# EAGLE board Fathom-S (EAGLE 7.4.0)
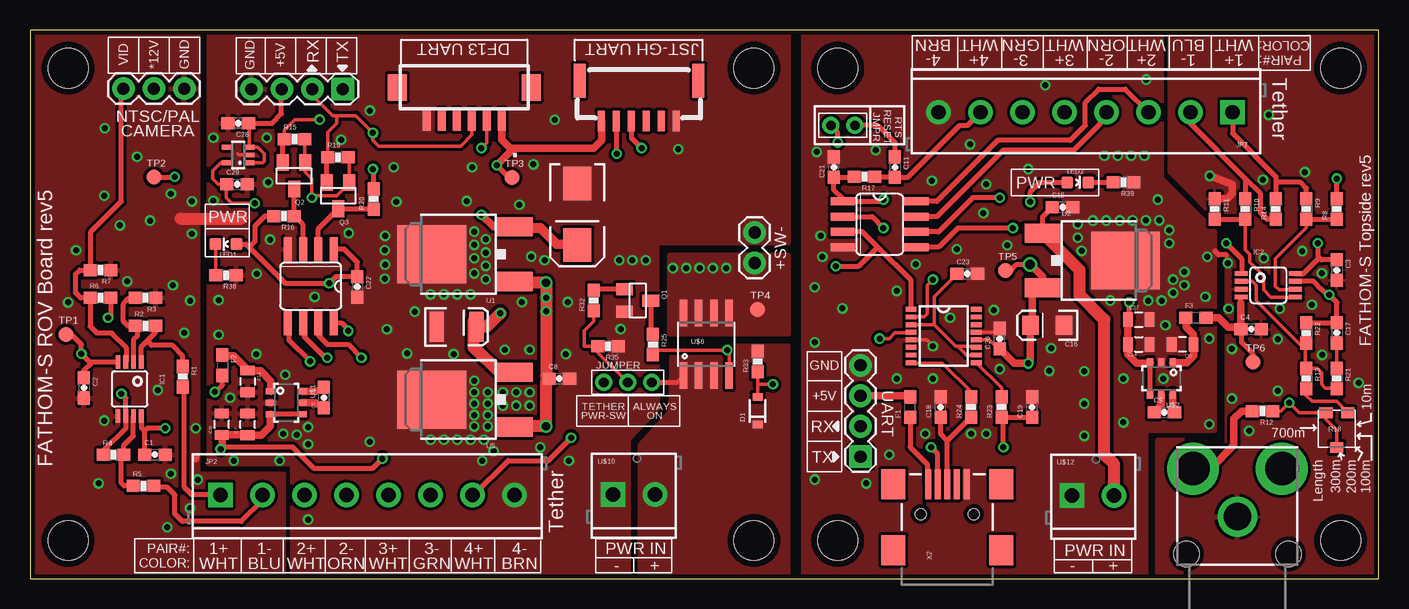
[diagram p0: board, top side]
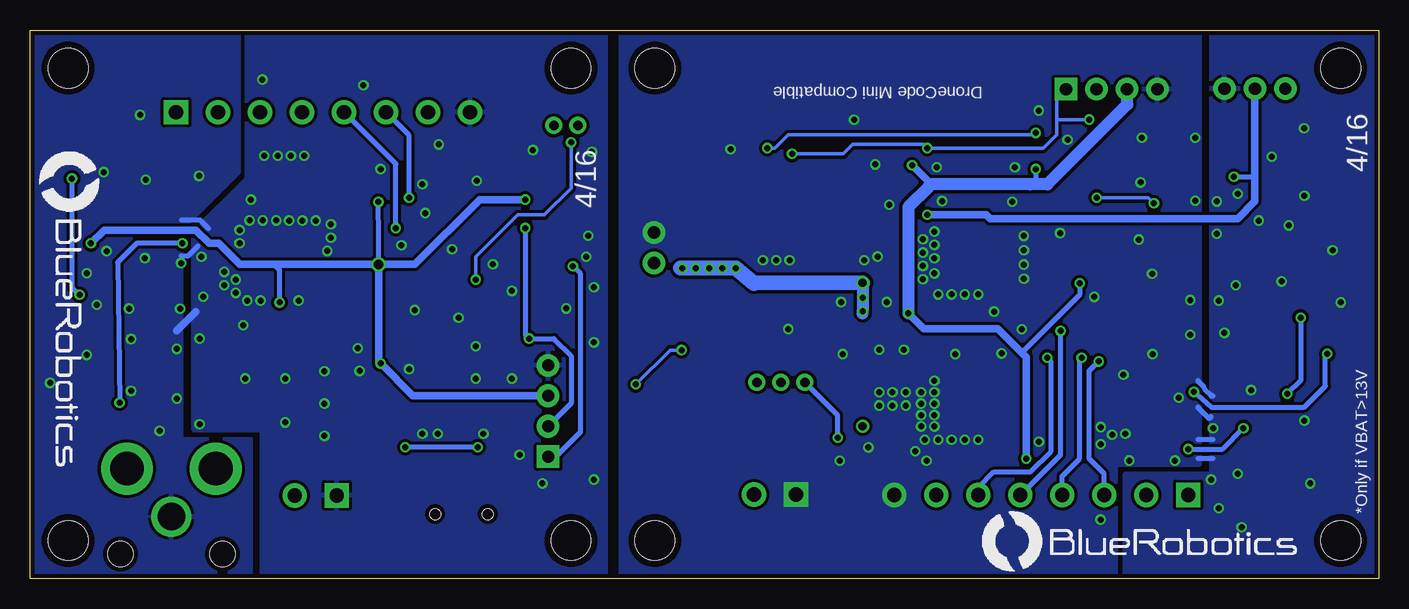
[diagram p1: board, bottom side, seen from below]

Size 112.39 x 45.72 mm. Coordinates in mm from the lower left corner, seen from the top.
Outline: 0,0 112.39,0 112.39,45.72 0,45.72 0,0
Copper layers (1*16): Top 0.0356mm / dielectric 1.5011mm / Bottom 0.0356mm
Design rules "OSH-Park *": minimum track width 6mil, minimum drill 13mil, track to track 6mil, track to pad 6mil, pad to pad 6mil, via to via 6mil, smd to smd 6mil, copper to edge 15mil, drill to drill 6mil, minimum pad ring 7mil, minimum via ring 7mil, stop-mask expansion 3mil, vias tented up to drill 30mil, thermal gap 10mil
Net classes: 1 power: width 0.254 mm

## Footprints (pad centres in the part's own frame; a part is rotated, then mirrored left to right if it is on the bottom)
0603-CAP = smd 1.1 x 1: 1 -0.85,0; 2 0.85,0
0805 = smd 0.8 x 1.2: 1 -0.9,0; 2 0.9,0
EIA3528 = smd 1.2 x 2.5: A 1.65,0; C -1.65,0
C2413 = smd 2.77 x 2.35: + 0,0; - 5.14,0
EIA3216 = smd 1.4 x 1.6: A 1.4,0; C -1.4,0
SOD-323 = smd 0.63 x 0.83: A 1.15,0; C -1.15,0
0603 = smd 1.1 x 1: 1 -0.85,0; 2 0.85,0
MSOP8 = smd 0.4 x 1.1: 1 -0.975,-2.25; 2 -0.325,-2.25; 3 0.325,-2.25; 4 0.975,-2.25; 5 0.975,2.25; 6 0.325,2.25; 7 -0.325,2.25; 8 -0.975,2.25
SO08 = smd 0.66 x 2.032: 1 -1.905,-3.073; 2 -0.635,-3.073; 3 0.635,-3.073; 4 1.905,-3.073; 5 1.905,3.073; 6 0.635,3.073; 7 -0.635,3.073; 8 -1.905,3.073
SSOP16 = smd 0.914 x 0.406: 1 -2.718,2.223; 2 -2.718,1.587; 3 -2.718,0.953; 4 -2.718,0.318; 5 -2.718,-0.318; 6 -2.718,-0.953; 7 -2.718,-1.587; 8 -2.718,-2.223; 9 2.718,-2.223; 10 2.718,-1.587; 11 2.718,-0.953; 12 2.718,-0.318; 13 2.718,0.318; 14 2.718,0.953; 15 2.718,1.587; 16 2.718,2.223
1X04 = drill 1.016 pad 1.88 square: 1 0,0 | drill 1.016 pad 1.88: 2 2.54,0; 3 5.08,0; 4 7.62,0
SCREWTERMINAL-3.5MM-8 = drill 1.2 pad 2.032 square: 1 0,0 | drill 1.2 pad 2.032: 2 3.5,0; 3 7,0; 4 10.5,0; 5 14,0; 6 17.5,0; 7 21,0; 8 24.5,0
1X03 = drill 1.016 pad 1.88: 1 0,0; 2 2.54,0; 3 5.08,0
1X02 = drill 1.016 pad 1.88: 1 0,0; 2 2.54,0
RCA = drill 2.8 pad 4.318: PIN 4,3.7; SWITCH 4,-3.7 | drill 2.3: SHELL 0,0 | hole 2.1: -3.1,4.25; -3.1,-4.25
LED-0603 = smd 1 x 1: A 0,-0.877; C 0,0.877
SOT23 = smd 1 x 1.4: 1 -0.95,-1.1; 2 0.95,-1.1; 3 0,1.1
0603-RES = smd 1.1 x 1: 1 -0.85,0; 2 0.85,0
TRIMPOT_TC33 = smd 1.1 x 0.9: 1 -0.91,-1.45; 2 0,1.45; 3 0.91,-1.45
STAND-OFF = hole 3.302: 0,0
B1,27 = smd 1.27 x 1.27: TP 0,0
DPAK = smd 1.6 x 3: 1 -2.28,-5.31; 3 2.28,-5.31 | smd 4.826 x 5.715: 4 0,1.588
SOT-23-6 = smd 0.51 x 0.8: 1 -0.95,-1.3; 2 0,-1.3; 3 0.95,-1.3; 4 0.95,1.3; 5 0,1.3; 6 -0.95,1.3
DF13C-6P-1.25V = smd 1.6 x 2.2: M$0 5.575,-1.8; M$1 -5.575,-1.8 | smd 0.7 x 1.8: P$1 -3.125,0.9; P$2 -1.875,0.9; P$3 -0.625,0.9; P$4 0.625,0.9; P$5 1.875,0.9; P$6 3.125,0.9
SO08' = smd 0.61 x 2.21: 1 -1.905,-2.616; 2 -0.635,-2.616; 3 0.635,-2.616; 4 1.905,-2.616; 5 1.905,2.616; 6 0.635,2.616; 7 -0.635,2.616; 8 -1.905,2.616
SCREWTERMINAL-3.5MM-2 = drill 1.2 pad 2.032 square: 1 0,0 | drill 1.2 pad 2.032: 2 3.5,0
JST-GH-TOP-6 = smd 0.6 x 1.7: 1 6.25,0; 2 5,0; 3 3.75,0; 4 2.5,0; 5 1.25,0; 6 0,0 | smd 1 x 2.8: MECH1 8.05,-3.35; MECH2 -1.85,-3.35
HEADER-2MM-3POS = drill 0.8 pad 1.422: P$1 0,0; P$2 2,0; P$3 4,0
SC70-5L = smd 0.4 x 0.8: 1 -0.65,-0.95; 2 0,-0.95; 3 0.65,-0.95; 4 0.65,0.95; 5 -0.65,0.95
HEADER-2MM-2POS = drill 0.8 pad 1.422: P$1 0,0; P$2 2,0
USB-MINIB = smd 2.5 x 0.5: D+ 2.5,0; D- 2.5,0.8; GND 2.5,-1.6; ID 2.5,-0.8; VBUS 2.5,1.6 | smd 2.5 x 2: GND@1 -3,-4.5; GND@2 -3,4.5; GND@3 2.5,4.5; GND@4 2.5,-4.5 | hole 0.9: 0,2.2; 0,-2.2

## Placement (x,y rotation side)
C1  0.1uF  [0603-CAP]  10.41,10.34 0 top
C2  0.1uF  [0603-CAP]  4.5,15.9 270 top
C3  0.1uF  [0603-CAP]  108.9,25.72 270 top
C4  0.1uF  [0603-CAP]  101.76,20.8 0 top
C5  1uF X5R 35V  [0603-CAP]  24.5,15.09 90 top
C6  10uF X5R 10V  [0805]  96.04,19.53 180 top
C7  10uF X5R 10V  [0805]  18.14,12.85 90 top
C8  0.1uF  [0603-CAP]  44.12,16.67 0 top
C9  1uF X5R 35V  [0603-CAP]  94.53,13.87 0 top
C10  47uF 10V  [EIA3528]  35.54,21 0 top
C11  1uF  [0603-CAP]  72.07,34.29 270 top
C12  10uF X5R 10V  [0805]  18.14,16.43 270 top
C13  33uF 20V  [C2413]  45.61,27.8 90 top
C14  10uF X5R 10V  [0805]  92.39,19.53 0 top
C15  0.1uF  [0603-CAP]  86.04,30.96 0 top
C16  10uF 16V  [EIA3216]  84.77,21.11 180 top
C17  68pF  [0603-CAP]  108.9,20.48 270 top
C18  47pF  [0603-CAP]  75.88,14.29 90 top
C19  47pF  [0603-CAP]  83.5,14.29 90 top
C20  0.1uF  [0603-CAP]  80.8,20 90 top
C21  0.1uF  [0603-CAP]  66.99,34.29 90 top
C22  0.1uF  [0603-CAP]  27.27,24.31 270 top
C23  0.1uF  [0603-CAP]  78.11,25.4 0 top
C26  10uF X5R 10V  [0805]  15.98,12.87 90 top
C27  10uF X5R 10V  [0805]  92.39,21.59 0 top
C28  1uF  [0603-CAP]  17.35,37.95 180 top
C29  1uF  [0603-CAP]  17.25,32.87 0 top
D1  16V  [SOD-323]  60.63,13.98 90 top
F1  500mA  [0603]  73.34,14.29 90 top
F2  500mA  [0603]  16.03,17.78 270 top
F3  500mA  [0603]  97.16,21.75 0 top
IC1  LMH6643  [MSOP8]  8.31,15.8 180 top
IC2  LMH6643  [MSOP8]  103.19,24.45 270 top
IC3  ST490AB  [SO08]  70.8,29.53 270 top
IC4  ST490AB  [SO08]  23.39,24.37 180 top
IC5  FT230XS  [SSOP16]  76.14,20.22 0 top
JP1  [1X04]  26.06,40.79 180 top
JP2  3.5MM SCREW  [SCREWTERMINAL-3.5MM-8]  15.88,6.99 0 top
JP3  0.1" HEADER  [1X03]  12.86,40.83 180 top
JP5  M02PTH  [1X02]  60.39,28.84 270 top
JP6  PJRAN1X1U04X  [RCA]  100.62,5.17 90 top
JP7  3.5MM SCREW  [SCREWTERMINAL-3.5MM-8]  100.22,38.87 180 top
JP15  0.1" HEADER  [1X04]  69.22,10.16 90 top
LED1  GREEN  [LED-0603]  16.33,27.88 90 top
LED2  GREEN  [LED-0603]  87.31,33.02 270 top
Q1  BC817-40W  [SOT23]  50.64,23.18 270 top
Q2  BSS138  [SOT23]  22,33.57 180 top
Q3  BSS138  [SOT23]  25.67,31.91 180 top
R1  43  [0603-RES]  12.73,16.83 270 top
R2  3K  [0603-RES]  9.61,21.06 0 top
R3  3K  [0603-RES]  9.64,23.39 180 top
R4  3K  [0603-RES]  6.97,10.31 0 top
R5  43  [0603-RES]  9.46,7.72 0 top
R6  1.5K  [0603-RES]  5.87,23.39 0 top
R7  75  [0603-RES]  5.87,25.72 180 top
R8  3K  [0603-RES]  108.9,30.8 90 top
R9  3K  [0603-RES]  106.36,30.8 270 top
R10  3K  [0603-RES]  101.28,30.8 270 top
R11  3K  [0603-RES]  98.74,30.8 270 top
R12  75  [0603-RES]  102.71,13.97 180 top
R13  1.5K  [0603-RES]  106.36,16.67 270 top
R14  86.6  [0603-RES]  103.82,30.8 90 top
R15  10K  [0603-RES]  22.03,36.63 0 top
R16  10K  [0603-RES]  21.16,30.22 180 top
R17  47K  [0603-RES]  69.53,33.5 180 top
R18  TC33X-2-102E  [TRIMPOT_TC33]  108.9,12.38 180 top
R19  10K  [0603-RES]  25.67,35.12 0 top
R20  10K  [0603-RES]  28.63,31.62 90 top
R21  3.9K  [0603-RES]  108.9,16.67 270 top
R22  3K  [0603-RES]  106.36,20.48 270 top
R23  27  [0603-RES]  80.96,14.29 90 top
R24  27  [0603-RES]  78.42,14.29 90 top
R25  10K  [0603-RES]  51.91,19.53 270 top
R32  47K  [0603-RES]  46.99,23.18 90 top
R33  5.1K  [0603-RES]  60.64,18.1 90 top
R35  47K  [0603-RES]  48.18,19.37 180 top
R38  330  [0603-RES]  16.32,25.29 180 top
R39  330  [0603-RES]  91.12,33.02 180 top
STANDOFF1  STAND-OFF  [STAND-OFF]  3.17,3.17 0 top
STANDOFF2  STAND-OFF  [STAND-OFF]  60.33,3.17 0 top
STANDOFF3  STAND-OFF  [STAND-OFF]  60.33,42.55 0 top
STANDOFF4  STAND-OFF  [STAND-OFF]  3.17,42.55 0 top
STANDOFF5  STAND-OFF  [STAND-OFF]  67.31,3.17 0 top
STANDOFF6  STAND-OFF  [STAND-OFF]  109.22,3.17 0 top
STANDOFF7  STAND-OFF  [STAND-OFF]  67.31,42.55 0 top
STANDOFF8  STAND-OFF  [STAND-OFF]  109.22,42.55 0 top
TP1  -5V  [B1,27]  2.98,20.35 0 top
TP2  12V  [B1,27]  10.32,33.45 0 top
TP3  5V  [B1,27]  40.16,33.42 0 top
TP4  VIN  [B1,27]  60.64,22.43 0 top
TP5  5V  [B1,27]  81.28,25.67 0 top
TP6  -5V  [B1,27]  101.92,18.05 0 top
U1  MC7812  [DPAK]  35.07,27.04 90 top
U2  MC7805  [DPAK]  89.69,26.51 270 top
U5  MC7805  [DPAK]  35.07,14.92 90 top
U$1  LM2776  [SOT-23-6]  21.36,14.66 270 top
U$2  LM2776  [SOT-23-6]  94.28,16.68 180 top
U$3  DF13-6P-1.25V  [DF13C-6P-1.25V]  36.19,39.14 180 top
U$4  LOGOFULL-M  [BR-FULL-LOGO-MEDIUM]  35.08,-0.79 0 bottom
U$5  LOGOBR-LOGO-MS-COPPER  [BR-LOGO-MEDIUM-SMALL-COPPER]  110.31,34.32 90 top
U$6  AO4407A  [SO08']  56.36,19.53 0 top
U$7  LOGOFULL-M  [BR-FULL-LOGO-MEDIUM]  113.03,37.62 270 bottom
U$9  LOGOBR-LOGO-MS  [BR-LOGO-MEDIUM-SMALL-COPPER]  51.1,33.56 270 top
U$10  M023.5MM  [SCREWTERMINAL-3.5MM-2]  48.58,7 0 top
U$11  JST-GH-6TOP-ENTRY  [JST-GH-TOP-6]  53.86,38.14 180 top
U$12  M023.5MM  [SCREWTERMINAL-3.5MM-2]  86.84,6.94 0 top
U$13  HEADER-33MM  [HEADER-2MM-3POS]  47.81,16.35 0 top
U$15  VREG-MIC5365  [SC70-5L]  17.34,35.3 90 top
U$16  HEADER-22MM  [HEADER-2MM-2POS]  68.74,37.77 180 top
X2  USBSMD  [USB-MINIB]  76.44,5.38 90 top

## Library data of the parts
C1-C10 C12 C14-C17 C26-C29 R1-R14 R21 R22 = SparkFun-Passives
C11 C18-C23 F1-F3 R15-R17 R19 R20 R23 R24 X2 = SparkFun
C13 IC1 IC2 JP6 TP1-TP6 U$4 U$5 U$7 U$9 U$13 U$15 U$16 = BlueRobotics-Main
D1 = SparkFun-DiscreteSemi; PROD_ID: DIO-11284; VALUE: 3.3V
IC3 IC4 = maxim; MF: MAXIM; MPN: MAX488CSA; OC_FARNELL: 3534170; OC_NEWARK: 34C3921
IC5 = ftdichip
JP1-JP3 JP5 JP7 JP15 U$10 U$12 = SparkFun-Connectors
LED1 LED2 = SparkFun-LED
Q1 U$6 = SparkFun-DiscreteSemi
Q2 Q3 = SparkFun-DiscreteSemi; PROD_ID: TRANS-00830
R18 STANDOFF1-STANDOFF8 = SparkFun-Electromechanical
R25 R32 R33 R35 R38 R39 = SparkFun-Resistors
U1 U2 U5 U$1 U$2 = BR-Eagle-Library
U$3 = con-hirose-df13
U$11 = BlueRobotics-JST-GH

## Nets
3.3V-ISO: C29.1 Q2.1 Q3.1 R15.2 R19.2 U$15.5
3V3OUT: C23.1 IC5.3 IC5.10 IC5.11
12V-ISO: C13.+ JP3.2 TP2.TP U1.3
-VCC: C4.1 F3.2 IC2.4 TP6.TP
-VCC-ISO: C2.1 F2.2 IC1.4 TP1.TP
-VCC-ISO-PRE: C12.1 F2.1 U$1.1
-VCC-PRE: C6.1 F3.1 U$2.1
CAMERA: IC1.3 JP3.3 R6.1 R7.2
GND: C3.2 C4.2 C6.2 C14.2 C15.2 C16.C C18.2 C19.2 C20.2 C21.2 C23.2 C27.2 IC2.3 IC3.4 IC5.5 IC5.13 JP6.SHELL JP7.8 JP15.4 R11.1 R39.1 U2.4 U$2.2 U$12.1 X2.GND
GND-ISO: C1.2 C2.2 C7.2 C8.2 C10.C C12.2 C13.- C22.2 C26.2 C28.2 C29.2 IC1.5 IC4.4 JP1.4 JP2.8 JP3.1 JP5.1 Q1.2 R3.1 R7.1 R35.1 R38.1 U1.4 U5.4 U$1.2 U$3.P$6 U$10.1 U$11.6 U$15.2
N$1: IC1.1 R1.1 R2.2
N$2: IC1.7 R4.2 R5.1
N$3: C9.1 U$2.5
N$4: C9.2 U$2.6
N$5: IC1.2 R2.1 R3.2
N$6: IC1.6 R4.1 R6.2
N$7: C11.1 U$16.P$1
N$8: IC2.5 R10.2 R11.2
N$9: IC2.6 R8.1 R9.2
N$10: C5.1 U$1.5
N$11: C5.2 U$1.6
N$12: R13.2 R18.1
N$14: C17.1 IC2.7 R8.2 R22.1
N$15: IC2.2 R13.1 R21.2 R22.2
N$16: C17.2 R21.1
N$17: IC2.1 R12.1 R18.2 R18.3
N$19: C19.1 R23.1 X2.D-
N$20: C18.1 R24.1 X2.D+
N$21: F1.1 X2.VBUS
N$22: IC5.8 R24.2
N$27: Q1.1 R32.2
N$28: D1.A R25.2 R33.1 U$6.4
N$29: IC5.9 R23.2
N$30: Q1.3 R25.1
N$31: LED1.C R38.2
N$32: LED2.C R39.2
ROV-BATT: D1.C R33.2 U$6.1 U$6.2 U$6.3 U$10.2 U$13.P$3
ROV-ON: JP2.7 U$13.P$1
ROV-ON-CTRL: C11.2 JP7.7 R17.1
ROV-ON-SELECT: R32.1 R35.2 U$13.P$2
ROV-RX: IC4.2 Q3.3 R20.1
ROV-TP1+: JP2.1 R1.2
ROV-TP1-: JP2.2 R5.2
ROV-TP2+: IC4.5 JP2.3
ROV-TP2-: IC4.6 JP2.4
ROV-TP3+: IC4.8 JP2.5
ROV-TP3-: IC4.7 JP2.6
ROV-TX: IC4.3 Q2.3 R16.1
ROV-VIN: C8.1 JP5.2 TP4.TP U1.1 U5.1 U$6.5 U$6.6 U$6.7 U$6.8
RTS: IC5.2 U$16.P$2
RX-3.3V: JP1.2 Q3.2 R19.1 U$3.P$3 U$11.3
RX-I: IC3.2 IC5.4 JP15.2
TOP-TP1+: JP7.1 R9.1 R14.2
TOP-TP1-: JP7.2 R10.1 R14.1
TOP-TP2+: IC3.8 JP7.3
TOP-TP2-: IC3.7 JP7.4
TOP-TP3+: IC3.5 JP7.5
TOP-TP3-: IC3.6 JP7.6
TOP-VIN: C15.1 U2.1 U$12.2
TX-3.3V: JP1.1 Q2.2 R15.1 U$3.P$2 U$11.2
TX-O: IC3.3 IC5.1 JP15.1
VCC: C3.1 C14.1 C16.A C20.1 C21.1 C27.1 F1.2 IC2.8 IC3.1 IC5.12 JP15.3 LED2.A R17.2 TP5.TP U2.3 U$2.3 U$2.4
VCC-ISO: C1.1 C7.1 C10.A C22.1 C26.1 C28.1 IC1.8 IC4.1 JP1.3 LED1.A R16.2 R20.2 TP3.TP U5.3 U$1.3 U$1.4 U$3.P$1 U$11.1 U$15.1 U$15.3
VIDEO-OUT: JP6.PIN R12.2

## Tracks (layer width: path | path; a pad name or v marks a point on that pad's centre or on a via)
3.3V-ISO  (via drill 0.5)
  Top 0.305: U$15.5 16.4,34.64 15.91,34.64 15.24,33.97 15.24,33.34 15.71,32.87 C29.1 16.35,32.82 16.35,31.75 16.83,31.27 v18.73,31.27 | R15.2 22.88,34.74 Q2.1 22.95,33.88 23.5,33.34 v23.5,31.75 23.81,31.91 25.56,31.91 26.62,32.97 Q3.1 26.62,35.02 R19.2
  Bottom 0.305: v23.5,31.75 19.21,31.75 v18.73,31.27
3V3OUT
  Top 0.305: IC5.3 75.35,21.17 | 75.35,21.17 77.15,19.37 77.31,19.37 | 77.31,19.37 78.75,19.37 IC5.11 | IC5.10 78.05,18.63 77.31,19.37 | 75.35,21.17 75.35,23.49 C23.1
12V-ISO  (via drill 0.5)
  Top 0.406: TP2.TP 12.02,33.45 v12.06,33.5
  Top 0.61: U1.3 38.63,29.32 v37.62,30.32
  Top 0.813: C13.+ 43.88,27.88 42.55,29.21 40.48,29.21 U1.3
  Bottom 0.406: v12.06,33.5 10.48,33.5 10.32,33.66
  Bottom 0.61: JP3.2 10.32,33.66 10.32,31.43 11.75,30 32.38,30 32.7,30.32 v37.62,30.32
-VCC
  Top 0.406: 100.89,22.94 100.89,23.42 IC2.4 | TP6.TP 101.92,18.73 100.97,19.68 100.97,20.74
  Top 0.61: C4.1 100.91,22.92 100.89,22.94 | 100.97,20.74 C4.1 | F3.2 99.06,21.75 99.85,20.95 100.75,20.95 C4.1
-VCC-ISO  (via drill 0.5)
  Top 0.406: v4.29,18.73 4.29,18.57 | IC1.4 5.18,18.05 | 5.18,18.05 4.97,18.05 v4.29,18.73 | C2.1 4.5,17.36 5.18,18.05 | v15.4,15.56 16.03,16.14 F2.2 | v4.29,18.73 4.29,19.53 3.65,20.16 3.18,20.16 TP1.TP
  Bottom 0.406: v4.29,18.73 4.45,18.57 4.45,16.03 6.19,14.29 13.97,14.29 v15.4,15.56
-VCC-ISO-PRE
  Top 0.61: U$1.1 20.06,16.45 19.21,17.3 18.17,17.3 C12.1 18.14,17.42 16.99,18.57 16.09,18.57 F2.1
-VCC-PRE
  Top 0.61: F3.1 96.36,21.69 96.36,20.95 96.94,20.37 C6.1 97,19.47 97,18.57 96.4,17.98 U$2.1
CAMERA
  Top 0.406: R7.2 4.13,25.72 3.81,25.4 3.81,23.81 4.23,23.39 R6.1 5.02,21.02 5.56,20.48 6.83,20.48 6.83,20.45 8,19.28 8,18.07 IC1.3 | 5.08,25.78 5.08,28.89 7.62,31.43 7.62,40.67 JP3.3
  Top 0.61: 5.08,25.78 R7.2
GND  (via drill 0.5)
  Top 0.305: IC5.5 74.71,19.9 v75.25,19.37 | IC5.13 80.97,20.54 C20.2
  Top 0.406: 99.69,26.99 99.06,26.99 98.74,27.3
  Top 0.61: R11.1 99.75,31.65 100.17,32.07 100.17,32.89 v98.3,33.56
  Bottom 0.406: 99.82,26.9 99.21,26.9 98.37,27.74 | 97.53,29.18 98.22,29.88 99.75,29.88
  Bottom 0.61: 100.17,20.64 98.58,22.23
  other vias: 80.33,22.38 75.25,16.67 94.61,21.11 94.46,16.67 91.12,13.02 106.83,22.82 100.16,15.01 110.72,16.31 103.23,38.64 102.75,33.24 95.25,24.92 94.93,29.05 93.98,31.59 106.01,27.3 107.66,25.45 84.93,17.3 79.69,12.06 72.23,16.67 72.23,23.97 65.41,24.29 65.56,35.56 73.82,26.19 76.68,21.75 85.09,19.21 90.81,29.84 87.31,28.42 81.44,27.78 66.04,26.83 98.11,26.83 91.12,16.67 74.61,12.06 65.41,8.26 83.19,34.13 93.03,41.59 84.61,41.12 70.48,35.72 80.8,17.46 65.88,28.57 65.41,19.68 69.69,7.94 71.6,10.32 107.67,18.64 101.59,12.31 106.24,33.88 97.95,23.5 78.42,12.06 103.97,19.96 103.97,15.65 100.16,19.14 99.89,22.49 99.81,26.3 102.81,26.71 104.14,22.5 90.01,23.18 93.19,23.18 98.27,20 91.88,29.85 92.99,29.85 94.1,29.85 89.69,29.84 88.58,29.84 87.31,29.53 87.63,27.3 94.93,27.94 95.25,23.81 94.3,23.18 96.2,24.45 96.2,25.56 98.27,12.86 89.53,35.24 90.65,35.24 91.76,35.24 92.87,35.24 79.45,30.47 77.23,27.45 75.16,33.17 78.34,36.18 87.86,17.29 87.86,14.59 87.86,11.89 79.7,32.87 67.7,22.51
  pour Top (isolate 0.254): 99.69,0 99.69,29.05 94.93,33.81 94.93,45.72 114.3,45.72 114.3,0
  pour Bottom (isolate 0.254): 99.69,-2.54 99.69,29.05 94.93,33.81 94.93,48.26 112.39,48.26 112.39,-2.54
  pour Bottom (isolate 0.254): 64.45,-2.54 93.03,-2.54 93.03,12.38 98.74,12.38 98.74,28.89 94.3,33.34 94.3,48.26 64.45,48.26
  pour Top (isolate 0.254, no thermals): 64.45,-1.27 93.03,-1.27 93.03,12.38 98.74,12.38 98.74,28.89 94.3,33.34 94.3,48.26 64.45,48.26
  pour Bottom (isolate 0.254): 93.98,-1.27 93.98,11.59 101.6,11.59 101.6,-1.27
  pour Top (isolate 0.254): 93.98,-2.54 93.98,11.59 101.6,11.59 101.6,-2.54
GND-ISO  (via drill 0.5)
  Top 0.305: U$15.2 17.4,35.3 17.3,35.4
  Top 0.61: 13.81,10.16 13.81,10
  Top 1.016: 12.54,30 17.62,30
  Bottom 0.406: 13.97,13.49 14.13,13.34 15.08,14.29 | 13.81,15.24 13.97,15.24 14.45,15.72 14.61,16.03 15.08,16.51 | 13.81,10 15.08,10 | 13.81,11.59 15.08,11.59
  other vias: 49.21,20.8 40.78,31.16 30.54,31.41 31.43,18.76 13.49,28.73 13.49,31.43 10.64,15.72 11.43,4.29 5.71,7.94 6.19,13.18 3.17,23.02 12.86,20.48 6.19,31.91 16.67,15.08 21.27,16.99 21.11,12.06 15.72,20.32 13.34,23.18 19.84,33.02 18.89,25.4 29.58,26.17 29.58,28.56 44.81,23.05 35.3,18.71 33.38,11.57 34.49,11.57 44.67,18.71 49.09,26.54 37.98,27.17 23.18,4.92 13.34,5.87 13.97,8.26 13.81,12.54 30.32,34.29 37.68,9.82 38.63,10.62 40.52,15.54 40.52,14.43 39.41,15.54 39.41,14.43 35.6,11.57 37.98,26.06 37.98,24.95 41,23.05 20.8,9.84 16.99,9.84 15.71,23.21 11.75,8.73 11.91,24.45 8.1,24.77 20,28.26 29.57,27.37 29.57,24.99 26.56,28.8 23.71,23.48 29.74,20.78 32.06,22.26 37.98,28.29 38.14,15.54 37.03,14.59 38.14,14.59 37.03,13.63 37.03,16.49 37.03,15.54 38.14,13.63 38.14,12.68 37.03,12.68 41.63,15.54 41.63,14.43 37.03,28.92 37.03,27.81 37.03,26.7 37.03,25.43 33.38,23.68 34.49,23.68 35.6,23.68 36.71,23.68 36.39,31.46 39.57,19.08 41.63,19.08 28.31,11.41 22.22,12 23.17,12.63 23.17,11.21 36.71,11.57 37.82,11.57 8.92,35.15 7.49,29.44 6.22,37.53 3.84,27.37 10,29.84 11.75,32.07 18.85,18.72 19.73,36.74 25.93,36.58 15.29,36.74 15.29,31.5 36.83,34.28 43.72,38.23 41.95,34.52 54.02,35.79 28.32,39.01 42.53,10.94 44.91,9.83 42.88,26.53 41.77,26.84 50.21,26.54 51.32,26.54
  pour Top (isolate 0.254): 12.7,-3.33 12.7,8.75 21.11,8.75 21.11,-3.33
  pour Bottom (isolate 0.254, no thermals): 21.91,45.72 63.18,45.72 63.18,-5.08 21.91,-5.08
  pour Top (isolate 0.254, no thermals): 21.91,48.26 63.18,48.26 63.18,27.94 52.23,27.94 52.23,25.08 52.26,23.34 52.26,14.18 49.85,11.64 49.85,-2.54 21.91,-2.54
  pour Top (isolate 0.254): 13.97,-1.27 -1.27,-1.27 -1.27,46.99 13.97,46.99
  pour Bottom (isolate 0.254): 13.97,-2.54 0,-2.54 0,48.26 13.97,48.26
  pour Bottom (isolate 0.254): 21.11,8.73 13.34,8.73 13.34,0 21.11,0
  pour Bottom (isolate 0.254): 14.92,9.53 14.92,46.99 27.29,46.99 27.29,9.53
  pour Top (isolate 0.254): 14.92,9.53 14.92,48.26 24.13,48.26 24.13,9.53
N$1
  Top 0.406: R1.1 12.72,18.59 11.89,19.43 10.13,19.43 9.75,19.81 | 10.21,20.8 R2.2 10.44,21.03 10.44,20.5 9.75,19.81 | IC1.1 9.28,19.34 9.75,19.81
N$2
  Top 0.406: R5.1 7.84,7.72 7.62,7.94 7.62,10.11 R4.2 7.82,11.1 8.61,11.89 8.61,13.53 IC1.7
N$3
  Top 0.61: U$2.5 94.28,14.48 C9.1
N$4
  Top 0.61: U$2.6 95.23,14.01 C9.2
N$5
  Top 0.406: R3.2 8.73,23.34 8.17,23.34 7.78,22.87 7.78,21.43 8.15,21.06 R2.1 8.94,20.88 8.94,20.22 8.61,19.89 8.61,18.07 IC1.2
N$6  (via drill 0.5)
  Top 0.406: R6.2 6.72,21.96 v6.51,21.75 | R4.1 6.12,10.69 8,12.57 8,13.53 IC1.6 7.98,15.04 v7.62,15.4
  Bottom 0.406: v6.51,21.75 6.51,16.51 v7.62,15.4
N$7
  Top 0.406: C11.1 72.07,36.35 70.64,37.78 68.76,37.78 U$16.P$1
N$8
  Top 0.305: R10.2 101.28,27.42 101.65,27.05 101.65,26.36 102.79,25.22 102.79,24.08 103.4,23.47 IC2.5
  Top 0.406: R11.2 R10.2
N$9
  Top 0.305: R9.2 106.36,29.25 103.78,26.67 103.78,24.38 104.09,24.08 105.39,24.08 IC2.6
  Top 0.406: R9.2 R8.1
N$10
  Top 0.61: U$1.5 23.76,14.66 C5.1
N$11
  Top 0.61: U$1.6 23.85,15.61 C5.2
N$12
  Top 0.305: R13.2 106.36,15.24 106.84,14.76 108.88,14.76 R18.1
  Top 0.406: 110.01,13.95 R18.1
N$14  (via drill 0.5)
  Top 0.406: R8.2 v108.9,33.34 | R22.1 C17.1 108.9,23.02 v108.27,23.65 108.1,23.65 107.62,24.13 | 107.63,24.13 107.62,24.13 | 107.62,24.13 106.98,24.77 IC2.7
  Bottom 0.406: v108.9,33.34 108.9,24.29 v108.27,23.65
N$15
  Top 0.305: IC2.2 101.87,24.77 102.18,24.46 102.18,23.16 105.82,19.53 106.26,19.53 106.26,17.62 R13.1 107.26,17.52 107.63,17.14 107.63,16.19 107.95,15.88 108.85,15.88 R21.2
  Top 0.406: 106.26,19.53 R22.2
N$16
  Top 0.305: C17.2 R21.1
N$17  (via drill 0.5)
  Top 0.305: R18.2 108.9,12.38 107.99,13.29 R18.3 105.76,13.83 v104.93,14.66 104.25,13.97 R12.1
  Top 0.406: v99.69,27.94 100.97,26.67 100.97,25.45 IC2.1 | 104.93,14.92 v104.93,14.66 | 108.88,10.95 R18.2
  Bottom 0.406: v99.69,27.94 103.5,27.94 105.09,26.35 v104.93,14.66
N$19  (via drill 0.5)
  Top 0.406: X2.D- 75.64,10.4 v75.09,10.95 | v81.12,10.95 81.12,13.28 R23.1 C19.1
  Bottom 0.406: v75.09,10.95 v81.12,10.95
N$20
  Top 0.406: X2.D+ 76.44,11.5 | 76.44,11.5 75.88,12.06 C18.1 | R24.1 78.38,13.44 76.44,11.5
N$21
  Top 0.406: F1.1 73.34,10.95 74.77,9.53 74.77,7.96 X2.VBUS
N$22
  Top 0.305: R24.2 78.42,15.56 76.04,17.94 73.48,17.94 IC5.8
N$27
  Top 0.406: Q1.1 47.25,24.13 R32.2
N$28  (via drill 0.5)
  Top 0.305: R33.1 60.64,16.19 | 60.64,16.19 60.64,15.47 D1.A | v61.91,16.19 60.64,16.19 | R25.2 52.28,19.05 v58.1,19.05 58.26,18.89 U$6.4
  Bottom 0.305: v58.1,19.05 59.05,19.05 v61.91,16.19
N$29
  Top 0.305: R23.2 80.96,15.89 IC5.9
N$30
  Top 0.406: Q1.3 51.74,20.39 R25.1
N$31
  Top 0.305: R38.2 15.47,27.86 LED1.C
N$32
  Top 0.406: LED2.C R39.2
ROV-BATT
  Top 0.305: 53.89,16.35 U$6.1
  Top 0.406: U$13.P$3 53.89,16.35
  pour Top (isolate 0.254, no thermals): 50.8,-2.54 63.18,-2.54 63.18,19.37 53.5,19.37 53.34,13.97 50.8,11.11
ROV-ON  (via drill 0.5)
  Top 0.406: JP2.7 36.99,6.99 39.85,9.84 43.18,9.84 v45.09,11.75
  Bottom 0.406: v45.09,11.75 45.09,13.62 U$13.P$1
ROV-ON-CTRL
  Top 0.406: JP7.7 78.14,37.78 77.47,37.78 73.13,33.44 C11.2 72.02,33.5 R17.1
ROV-ON-SELECT
  Top 0.305: R32.1 46.99,21.43 46.2,20.64 46.2,19.37 R35.2 47.33,18.84 U$13.P$2
ROV-RX
  Top 0.406: IC4.2 24.03,29.17 Q3.3 28.58,30.82 R20.1
ROV-TP1+
  Top 0.406: JP2.1 13.49,6.99 12.86,7.62 12.86,15.84 R1.2
ROV-TP1-
  Top 0.406: JP2.2 19.38,6.52 17.62,4.76 12.7,4.76 12.06,5.4 12.06,6.99 11.43,7.62 10.41,7.62 R5.2
ROV-TP2+  (via drill 0.5)
  Top 0.406: v23.34,18.1 21.59,19.84 21.59,21.2 IC4.5
  Bottom 0.406: JP2.3 22.88,8.75 24.13,10 24.13,17.3 v23.34,18.1
ROV-TP2-  (via drill 0.5)
  Top 0.406: v24.77,18.41 24.61,18.41 22.86,20.16 22.86,21.2 IC4.6
  Bottom 0.406: JP2.4 26.38,8.55 24.92,10 24.92,18.26 v24.77,18.41
ROV-TP3+  (via drill 0.5)
  Top 0.406: v26.51,20.64 26.51,20.8 26.04,21.27 25.33,21.27 IC4.8
  Bottom 0.406: JP2.5 29.84,6.99 26.51,10.32 v26.51,20.64
ROV-TP3-  (via drill 0.5)
  Top 0.406: IC4.7 24.03,20.26 24.77,19.53 26.51,19.53 v27.62,18.41
  Bottom 0.406: JP2.6 33.38,7.58 32.07,8.89 29.05,8.89 27.3,10.64 27.3,18.1 v27.62,18.41
ROV-TX
  Top 0.406: IC4.3 22.76,29.47 R16.1 22.01,32.46 Q2.3
ROV-VIN  (via drill 0.5, 0.7)
  Top 1.016: U1.1 40.48,24.65 v43.01,24.65 43.01,16.93 C8.1 43.01,16.41 v43.01,12.7 40.44,12.7 U5.1 | v43.01,23.42 v43.01,22.28
  Bottom 1.016: v43.01,24.65 v43.01,22.27 | 43.01,22.11 v43.01,22.27 | v43.01,22.27 v43.01,22.28
  Bottom 1.27: v43.01,24.65 52.07,24.61 v53.58,25.88 58.18,25.88
  other vias: 54.69,25.88 55.8,25.88 56.91,25.88 58.02,25.88
  pour Top (isolate 0.254, no thermals): 53.32,20.36 53.32,27 63.18,26.99 63.18,20.32
RTS  (via drill 0.5)
  Top 0.305: IC5.2 74.51,21.81 74.77,22.07 74.77,24.45 v75.25,24.92
  Top 0.406: v67.31,36.35 67.31,37.19 U$16.P$2
  Bottom 0.305: v75.25,24.92 75.25,26.83 71.75,30.32 69.53,30.32 67.31,32.54 v67.31,36.35
RX-3.3V  (via drill 0.5)
  Top 0.305: U$3.P$3 36.81,36.97 35.88,36.04 29.05,36.04 28.57,36.51 v28.57,37.15 27.15,38.58 25.56,38.58 | JP1.2 23.52,40.29 25.24,38.58 25.56,38.58 | R19.1 24.82,37.2 25.56,37.94 25.56,38.58
  Top 0.406: U$11.3 50.11,36.73 v50.96,35.88 | Q3.2 24.72,35.03 R19.1
  Bottom 0.305: v50.96,35.88 50.32,35.88 49.21,36.99 28.73,36.99 v28.57,37.15
RX-I  (via drill 0.5)
  Top 0.305: v70.8,20 71.6,20 72.07,20.48 73.36,20.48 IC5.4
  Top 0.406: IC3.2 70.17,30.16 v71.12,29.21
  Bottom 0.406: v71.12,29.21 71.12,20.32 v70.8,20 68.74,20 67.31,18.57 67.31,14.61 JP15.2
TOP-TP1+
  Top 0.406: JP7.1 100.22,37.1 103.82,33.5 103.82,33.18 | 103.82,33.18 R14.2 | R9.1 106.36,32.54 105.89,33.02 103.98,33.02 103.82,33.18
TOP-TP1-
  Top 0.406: JP7.2 96.72,37.9 101.28,33.34 | 101.28,33.34 R10.1 | R14.1 103.08,29.95 102.55,30.48 102.55,32.07 101.28,33.34
TOP-TP2+
  Top 0.406: JP7.3 91.29,40.8 89.06,40.8 87.95,39.69 87.95,37.78 86.68,36.51 80.64,36.51 75.56,31.43 IC3.8
TOP-TP2-
  Top 0.406: JP7.4 89.22,38.36 89.22,37.94 87,35.72 81.12,35.72 75.56,30.16 IC3.7
  Bottom 0.406: 89.69,38.84 JP7.4
TOP-TP3+  (via drill 0.5)
  Top 0.406: v81.92,29.21 77.31,29.21 75.72,27.62 IC3.5
  Bottom 0.406: JP7.5 81.92,34.56 v81.92,29.21
TOP-TP3-  (via drill 0.5)
  Top 0.406: v80.8,31.75 78.58,31.75 75.72,28.89 IC3.6
  Bottom 0.406: JP7.6 80.8,36.95 v80.8,31.75
TOP-VIN
  Top 0.406: U2.1 84.38,30.15 C15.1
  Top 1.016: U2.1 87.47,25.7 87.47,23.65 89.53,21.59 89.53,10.32 90.34,9.52 U$12.2
TX-3.3V  (via drill 0.5)
  Top 0.305: U$3.P$2 38.06,36.32 v37.62,35.88 | R15.1 21.18,37.37 22.07,38.26 v24.13,38.26
  Top 0.406: U$11.2 48.86,35.44 v48.9,35.4 | Q2.2 21.05,36.5 R15.1
  Bottom 0.305: v48.9,35.4 44.61,35.4 43.81,36.2 37.94,36.2 v37.62,35.88 27.94,35.88 26.83,36.99 26.83,38.1 | 26.83,38.1 26.83,40.03 JP1.1 | v24.13,38.26 26.67,38.26 26.83,38.1
TX-O  (via drill 0.5)
  Top 0.406: IC5.1 73.42,24.85 70.64,27.62 | 70.64,27.62 69.37,28.89 IC3.3 | v67.15,26.04 69.06,26.04 70.64,27.62
  Bottom 0.406: JP15.1 68.58,10.16 66.52,12.22 66.52,25.4 v67.15,26.04
VCC  (via drill 0.5, 0.8)
  Top 0.305: IC5.12 79.95,19.9 80.64,19.21 81.22,19.21 C20.1
  Top 0.406: C3.1 107.63,26.57 107.45,26.75 | v107.31,27.94 107.31,26.89 107.45,26.75 | v71.12,31.59 71.28,31.43 IC3.1 67.73,31.65 66.99,32.38 C21.1 68.63,33.44 R17.2 | U$2.4 U$2.3 | IC2.8 106.12,25.42 107.45,26.75 | 91.6,21.7 v91.6,23.02 | v83.36,31.39 83.36,32.24 84.14,33.02 LED2.A | TP5.TP 81.71,25.67 82.23,26.19 v83.34,26.19
  Top 0.61: JP15.3 72.89,15.24 F1.2 | C20.1 82.02,17.94 v83.19,17.94 83.37,18.13 C16.A 83.37,20.98 | 91.44,19.47 C14.1 | 91.6,19.63 C14.1 | 91.6,21.7 C27.1 C14.1 | C14.1 91.49,18.68 92.23,17.94 93.29,17.94 U$2.3 | U2.3 84.38,25.15 v83.34,26.19 | 83.5,24.13 83.5,21.11 83.37,20.98 | 83.37,20.98 83.34,20.95
  Bottom 0.406: v83.34,26.19 83.34,28.36 v83.36,31.39 | v91.6,23.02 91.6,25.72 92.08,26.19
  Bottom 0.61: v107.31,27.94 106.2,29.05 98.58,29.05 97.47,27.94 96.68,27.94 94.93,26.19 92.08,26.19 v83.34,26.19 | JP15.3 80.49,15.24 v83.19,17.94 83.34,18.1 v83.34,26.19 | v83.34,26.19 80.33,26.19 74.93,31.59 v71.12,31.59
VCC-ISO  (via drill 0.5)
  Top 0.305: U$15.1 19.41,34.65 19.53,34.77 19.53,35.4 18.97,35.95 U$15.3 18.29,37.86 C28.1
  Top 0.406: U$1.4 U$1.3 | C1.1 9.56,12.3 | 9.56,12.3 9.3,12.57 9.3,13.53 IC1.8 | v11.27,12.54 9.8,12.54 9.56,12.3 | 16.03,10.95 21.91,10.95 23.65,9.21 28.57,9.21 v29.37,10 | C28.1 20.17,37.95 20.95,38.73 20.95,40.77 JP1.3 | IC4.1 25.31,27.46 26.19,27.46 27.27,26.38 C22.1 25.48,25.16 v24.92,24.61 21.27,24.61 18.26,27.62 | R20.2 28.63,34.08 v28.57,34.13 | LED1.A 18,27.88 18.26,27.62 | R16.2 19.58,30.22 18.73,29.37 18.73,28.1 18.26,27.62 | TP3.TP 39.92,33.42 v38.89,34.45
  Top 0.61: U5.3 39.14,17.2 | 36.97,21.45 C10.A | 18.15,11.96 C7.1 | C7.1 18.12,11.97 C26.1 16.03,11.91 16.03,10.95 v15.88,10.79 | C7.1 19.25,11.95 20,12.7 20,13.65 U$1.3 | U$3.P$1 39.31,36.57 40.01,35.88 40.32,35.88 | 40.32,35.88 46.99,35.88 47.62,36.51 47.62,38.13 U$11.1 | v38.89,34.45 40.32,35.88
  Top 1.016: v39.2,22.11 38.05,21 C10.A | 39.14,17.2 36.97,19.26 36.97,21.45
  Bottom 0.406: 39.35,22.27 v39.2,22.11 | v15.88,10.79 13.02,10.79 v11.27,12.54 | v28.57,34.13 28.57,33.34 29.05,32.86 | v24.92,24.61 24.92,23.65 29.74,18.84
  Bottom 0.61: v39.2,22.11 37.92,20.84 31.75,20.84 29.74,18.84 29.37,18.46 v29.37,10 | 37.47,32.7 37.47,33.02 v38.89,34.45
  Bottom 1.016: v39.2,22.11 39.2,30.97 37.47,32.7 37.31,32.86 29.05,32.86 27.62,32.86 20.95,39.53 20.95,40.77 JP1.3
VIDEO-OUT
  Top 0.61: JP6.PIN 98.38,9.16 100.33,11.11 100.33,13.34 100.97,13.97 R12.2

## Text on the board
tPlace: DF13 UART | JST-GH UART | VID | *12V | GND | GND | +5V | RX | TX | 4- / BRN | 4+ / WHT | 3- / GRN | 3+ / WHT | 2- / ORN | 2+ / WHT | 1- / BLU | 1+ / WHT | PAIR#: / COLOR: | Tether | NTSC/PAL / CAMERA | RTS / RESET / JMPR | PWR | PWR | +SW- | FATHOM-S Topside rev5 | GND | JUMPER | UART | 10m | +5V | TETHER / PWR-SW | ALWAYS / ON | RX | 700m | TX | Length | 300m | 200m | 100m | FATHOM-S ROV Board rev5 | Tether | PWR IN | PAIR#: / COLOR: | 1+ / WHT | 1- / BLU | 2+ / WHT | 2- / ORN | 3+ / WHT | 3- / GRN | 4+ / WHT | 4- / BRN | PWR IN | - | + | - | +
bPlace: DroneCode Mini Compatible | 4/16 | 4/16 | *Only if VBAT>13V
Reference: <-- VSCORE

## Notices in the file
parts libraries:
SparkFun-Passives: Licensing: Creative Commons ShareAlike 4.0 International - https://creativecommons.org/licenses/by-sa/4.0
